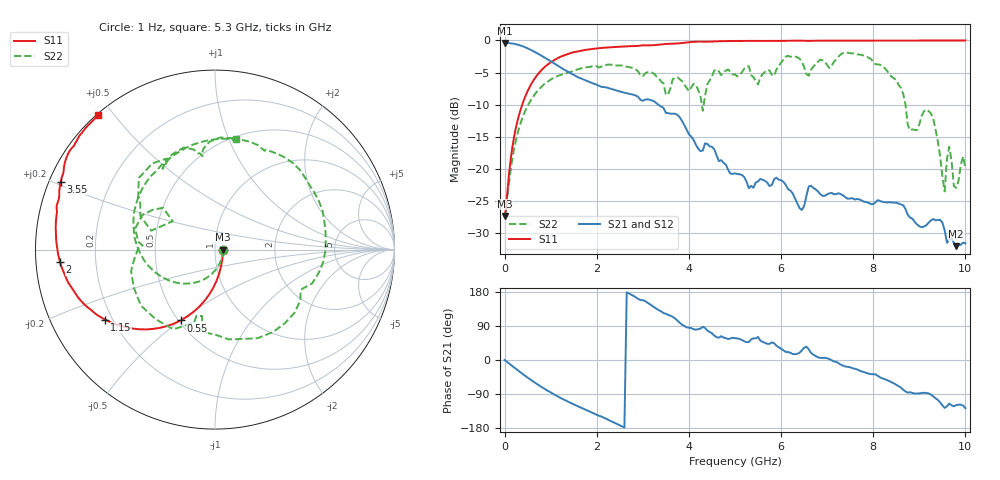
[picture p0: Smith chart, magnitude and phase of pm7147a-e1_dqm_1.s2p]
# GHz S DB R 50
! S-Parameters data
! Freq  dbS11  angS11  dbS21  angS21  dbS12  angS12  dbS22  angS22
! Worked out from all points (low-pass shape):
!   279 points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, 1 Hz to 10 GHz, reference 50 ohm
!   highest |S21| = -0.38 dB at 1.6 Hz (marker M1); lowest = -32.0 dB at 9.8 GHz (marker M2)
!   |S21| within 3 dB of the highest: start of sweep to 1.033 GHz
!   lowest |S11| = -27.3 dB at 2 Hz (marker M3), VSWR 1.09, Z = 54.5 - j1.25e-07 ohm
!   |S11| at or under -10 dB: start of sweep to 381.8 MHz
!   |S22| runs from -27.3 to -1.9 dB; largest |S21 - S12| = 1.2e-12
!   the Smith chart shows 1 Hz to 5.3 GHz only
!   S11 on the Smith chart (normalised r, x): 1 Hz: 1.09, -0.00; 550 MHz: 0.51, -0.50; 1.15 GHz: 0.17, -0.28; 2 GHz: 0.07, -0.04; 3.55 GHz: 0.03, +0.21; 5.3 GHz: 0.00, +0.46
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1e-09  -27.27 -0.0  -0.38 -0.0  -0.38 -0.0  -27.27 -0.0
1.6e-09  -27.27 -0.0  -0.38 -0.0  -0.38 -0.0  -27.27 -0.0
2e-09  -27.27 -0.0  -0.38 -0.0  -0.38 -0.0  -27.27 -0.0
0.55  -7.16 -115.9  -1.41 -50.8  -1.41 -50.8  -9.52 -153.0
1.15  -2.77 -147.6  -3.90 -96.0  -3.90 -96.0  -5.55 140.3
1.7  -1.54 -167.3  -6.04 -127.9  -6.04 -127.9  -4.29 93.4
2  -1.25 -175.5  -6.89 -144.5  -6.89 -144.5  -4.02 67.6
2.75  -0.90 168.7  -8.36 172.4  -8.36 172.4  -4.22 -0.6
3.35  -0.66 159.3  -10.06 131.2  -10.06 131.2  -5.92 -81.5
3.55  -0.55 156.2  -11.30 119.1  -11.30 119.1  -8.35 -105.7
3.85  -0.41 152.0  -12.51 93.3  -12.51 93.3  -6.33 -165.7
5.05  -0.10 134.2  -20.78 57.1  -20.78 57.1  -5.59 97.6
5.3  -0.07 131.0  -22.96 47.5  -22.96 47.5  -4.01 79.2
6.7  -0.06 115.8  -22.92 14.1  -22.92 14.1  -4.10 44.7
7.55  -0.04 107.9  -24.53 -21.7  -24.53 -21.7  -2.01 7.0
8.35  -0.03 101.3  -25.15 -55.8  -25.15 -55.8  -5.24 -43.9
8.8  -0.02 97.9  -27.56 -85.0  -27.56 -85.0  -13.99 -58.1
9.25  -0.02 94.6  -28.00 -91.2  -28.00 -91.2  -11.32 -71.2
9.55  -0.02 92.6  -29.51 -126.6  -29.51 -126.6  -23.47 -82.4
9.65  -0.02 91.9  -30.90 -115.1  -30.90 -115.1  -16.52 -99.1
9.8  -0.01 90.9  -31.98 -119.1  -31.98 -119.1  -22.92 -115.1
10  -0.01 89.6  -31.54 -127.0  -31.54 -127.0  -19.71 -162.9
